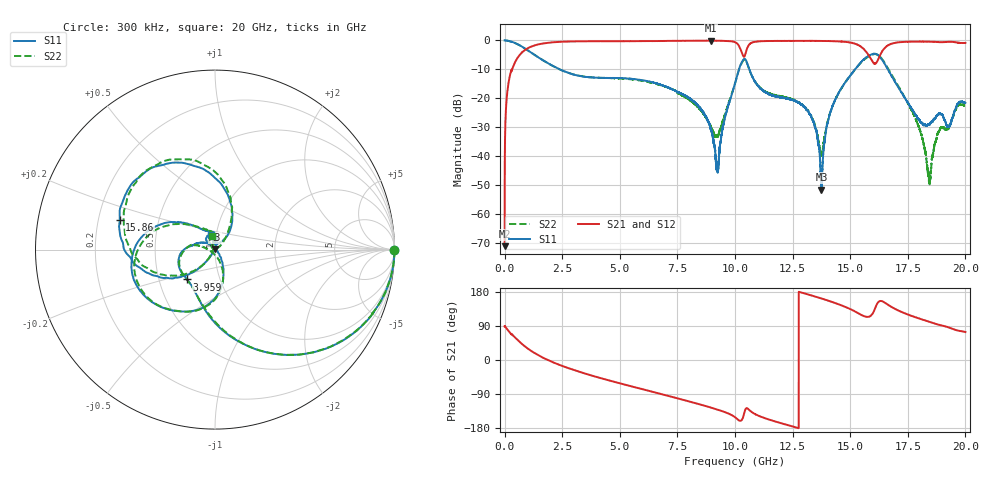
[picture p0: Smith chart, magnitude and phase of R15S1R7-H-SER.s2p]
!{R15S1R7}
!Johanson Technology Inc.
!www.johansontechnology.com
!Test Board Conditions:
!Substrate Type  RO4350B
!Substrate Thickness  20 mil
!Substrate Dk  3.66
!TL Type: GCPW
!TL Trace Width  34 mil
!TL Gap  10 mil
!Electrode orientation  Horizontal
!DUT TOPOLOGY	SERIES
!Mounting Pad LxW  26x52 mil
! Created Sat Feb  6 12:17:25 2021
# hz S ma R 50
! 2 Port Network Data from SP1.SP block
! freq  magS11  angS11  magS21  angS21  magS12  angS12  magS22  angS22
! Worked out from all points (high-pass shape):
!   20001 points, 300 kHz to 20 GHz, reference 50 ohm
!   highest |S21| = -0.07 dB at 8.957 GHz (marker M1); lowest = -71.0 dB at 300 kHz (marker M2)
!   |S21| within 3 dB of the highest: 926.5 MHz to 10.24 GHz (9.314 GHz wide, 167 % of centre); 10.51 GHz to 15.6 GHz (5.092 GHz wide, 39 % of centre)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
!   lowest |S11| = -51.5 dB at 13.75 GHz (marker M3), VSWR 1.01, Z = 49.7 + j0.0896 ohm
!   |S11| at or under -10 dB: 2.393 GHz to 10.17 GHz (7.777 GHz wide, 124 % of centre); 10.62 GHz to 15.21 GHz (4.591 GHz wide, 35.5 % of centre); 16.64 GHz to end of sweep
!   |S22| runs from -49.7 to 0.0 dB; largest |S21 - S12| = 0.014
!   S11 on the Smith chart (normalised r, x): 300 kHz: open; 3.959 GHz: 0.69, -0.24; 15.86 GHz: 0.29, +0.14; 20 GHz: 0.95, +0.15
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300000  1 -0.3  0.0002805 88.9  0.0002301 93.5  0.9959 -0.2
1.293e8  0.9892 -9.8  0.1413 79.9  0.1419 79.9  0.9889 -9.8
4.843e8  0.8933 -32.4  0.4451 57.3  0.4461 57.4  0.8919 -32.3
1.6313e9  0.4648 -83.1  0.8815 7.2  0.8822 7.1  0.4642 -82.4
3.3343e9  0.2409 -122.4  0.9663 -32.7  0.9656 -32.8  0.2423 -122.4
3.9593e9  0.228 -133.3  0.9698 -44.2  0.9698 -44.2  0.2283 -134.3
6.6673e9  0.1773 -178.8  0.9775 -87.8  0.9789 -87.8  0.1745 -177.4
8.9573e9  0.02815 126.8  0.9923 -125.6  0.9909 -125.6  0.0318 -171.4
9.2483e9  0.005486 28.4  0.9894 -131.0  0.988 -131.1  0.02275 -114.4
1.00003e10  0.18 -75.6  0.9343 -151.0  0.9347 -150.9  0.1816 -75.9
1.04263e10  0.4808 -163.7  0.5461 -134.5  0.5468 -134.6  0.4688 -159.4
1.12703e10  0.1319 121.9  0.974 -152.9  0.9743 -153.0  0.1341 119.0
1.33343e10  0.04535 78.6  0.983 170.0  0.9844 170.1  0.04692 94.1
1.37533e10  0.002668 160.3  0.9821 162.3  0.9819 162.4  0.01067 171.2
1.43093e10  0.08681 -126.7  0.9718 151.1  0.9734 151.2  0.08678 -127.0
1.58603e10  0.5552 162.9  0.5108 115.3  0.5104 115.0  0.548 158.1
1.66673e10  0.2994 74.9  0.8372 144.7  0.8326 145.4  0.3169 75.2
1.79403e10  0.04496 57.4  0.9555 110.5  0.9592 110.7  0.03474 36.0
1.84203e10  0.03532 94.2  0.9524 101.0  0.9533 100.8  0.004068 83.4
1.88703e10  0.05478 97.4  0.9338 92.7  0.9351 92.6  0.02718 132.9
1.92693e10  0.03321 112.9  0.9479 85.9  0.9492 86.2  0.03074 121.9
2e10  0.08323 105.2  0.9046 73.8  0.9015 73.6  0.07581 101.2
